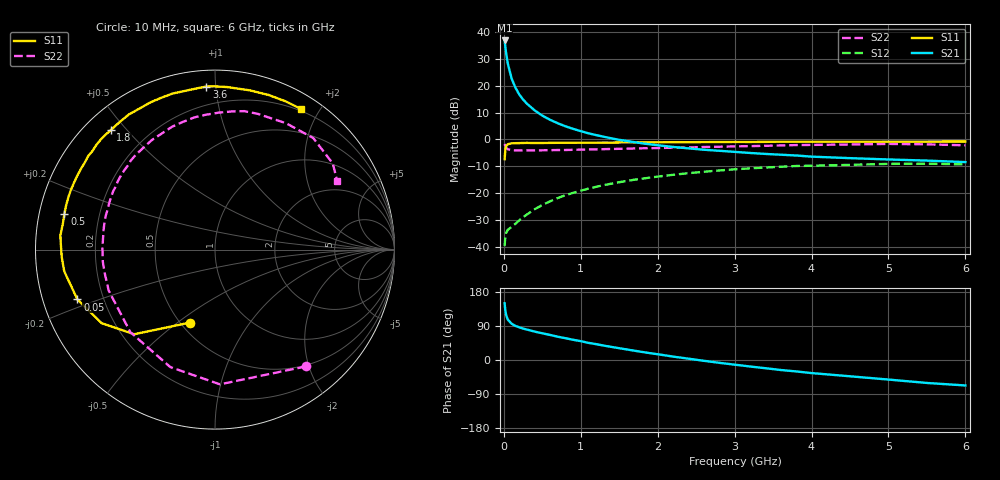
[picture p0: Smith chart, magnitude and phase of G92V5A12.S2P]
! SIEMENS Small Signal Semiconductors
! BFG235
! Si NPN RF Bipolar Junction Transistor in SOT223
! VCE = 2.5 V  IC = 120 mA
! Common Emitter S-Parameters:  July  1994
# GHz  S  MA  R  50
!  f  S11  S21  S12  S22
! GHz  MAG  ANG  MAG  ANG  MAG  ANG  MAG  ANG
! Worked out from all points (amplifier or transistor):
!   40 points, 10 MHz to 6 GHz, reference 50 ohm
!   highest |S21| = 36.7 dB at 10 MHz (marker M1)
!   |S21| within 3 dB of that: start of sweep to 22.59 MHz
!   unconditionally stable (mu >= 1): 448 MHz to 1.55 GHz
!   at 200 MHz: K = 0.80, MSG = 23.4 dB, |S12| = -30.0 dB
!   at 1.5 GHz: K = 1.00, MAG = 7.5 dB, |S12| = -15.8 dB
!   at 6 GHz: K = 0.91, MSG = 0.4 dB, |S12| = -9.2 dB
!   S11 on the Smith chart (normalised r, x): 10 MHz: 0.56, -0.56; 50 MHz: 0.10, -0.17; 500 MHz: 0.08, +0.12; 1.8 GHz: 0.07, +0.45; 3.6 GHz: 0.09, +0.94; 6 GHz: 0.18, +1.76
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0.01  0.4297 -108.9  68.74 149.8  0.0105 60.3  0.8247 -52.1
0.02  0.6523 -133.7  52.11 130.3  0.0161 45.3  0.7511 -87.9
0.03  0.7528 -147.0  40.02 118.8  0.0187 37.6  0.7004 -110.8
0.05  0.8153 -160.1  26.17 107.0  0.0209 32.2  0.6588 -135.7
0.1  0.8486 -171.8  13.68 95.8  0.024 35.4  0.6348 -158.9
0.15  0.8552 -177.4  9.171 90.0  0.0273 41.4  0.6284 -168.4
0.2  0.8571 179.7  6.858 86.3  0.0316 46.0  0.6288 -173.9
0.25  0.8613 176.9  5.526 82.9  0.0362 49.7  0.6267 -177.7
0.3  0.8651 174.7  4.615 80.3  0.0406 53.0  0.6275 179.0
0.4  0.8597 170.3  3.475 75.0  0.0508 55.7  0.627 174.2
0.5  0.862 166.8  2.775 70.4  0.061 57.1  0.6305 170.1
0.7  0.8676 160.2  2.005 61.5  0.082 56.6  0.6373 162.8
0.9  0.8693 154.8  1.576 53.4  0.1023 53.5  0.6436 156.5
1.1  0.8723 148.3  1.302 45.2  0.1227 50.2  0.6537 150.3
1.4  0.8762 141.1  1.049 34.5  0.1517 44.2  0.6673 141.7
1.8  0.8831 131.2  0.848 21.2  0.188 35.4  0.6871 130.6
2.2  0.8928 122.5  0.728 9.0  0.2212 26.4  0.7048 119.8
3.2  0.8998 101.2  0.563 -17.1  0.2911 3.2  0.7532 93.8
3.6  0.9099 93.0  0.522 -26.4  0.3121 -6.6  0.7759 82.9
4.5  0.9082 77.7  0.451 -43.0  0.3387 -26.1  0.8078 60.6
5.5  0.9149 64.6  0.406 -60.6  0.3559 -47.6  0.8128 36.2
6  0.9183 58.7  0.381 -67.2  0.3461 -55.7  0.7804 29.1
